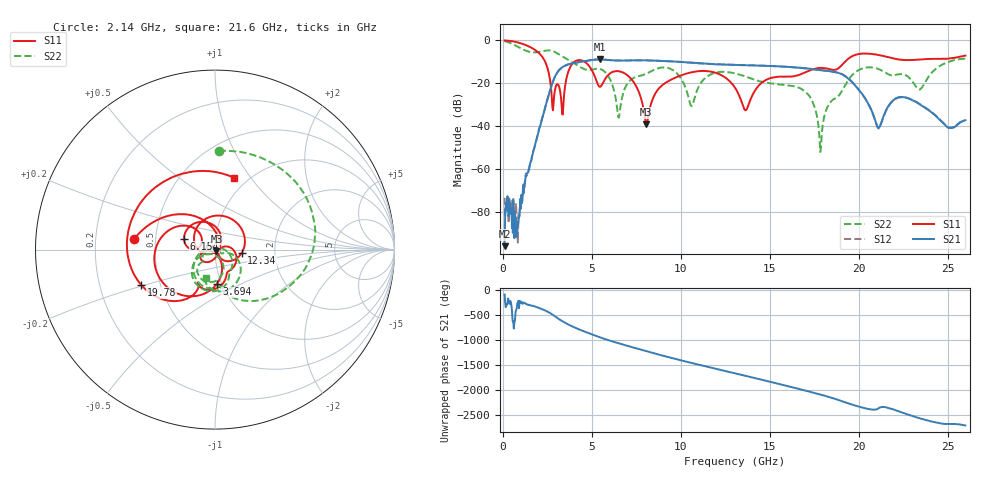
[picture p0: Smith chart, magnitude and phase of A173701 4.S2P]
!  2-Port S-parameters saved by WinCal
! VAR MeasName=S-Parameters (CALIBRATED_DATA) read from VNA (N5245A)
! VAR MeasDate=2017-6-7 10:28:41
! VAR NAME=A173701 4
! VAR FILENAME=A173701 4.S2P
! VAR DATE=2017-6-7 10:28:41
! VAR PHYS_PORTS=1,2
# Hz S DB R 50
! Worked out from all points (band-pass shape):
!   801 points, 100 MHz to 26 GHz, reference 50 ohm
!   highest |S21| = -8.86 dB at 5.442 GHz (marker M1); lowest = -96.1 dB at 100 MHz (marker M2)
!   |S21| within 3 dB of the highest: 3.481 GHz to 14.81 GHz (11.32 GHz wide, 124 % of centre)
!   lowest |S11| = -39.2 dB at 8.064 GHz (marker M3), VSWR 1.02, Z = 50.8 - j0.768 ohm
!   |S11| at or under -10 dB: 2.38 GHz to 4.019 GHz (1.639 GHz wide, 51.2 % of centre); 4.605 GHz to 19.23 GHz (14.62 GHz wide, 123 % of centre)
!   |S22| runs from -52.1 to -0.3 dB; largest |S21 - S12| = 0.0043
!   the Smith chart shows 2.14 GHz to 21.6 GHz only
!   S11 on the Smith chart (normalised r, x): 2.14 GHz: 0.38, +0.06; 3.694 GHz: 0.94, -0.38; 6.154 GHz: 0.70, +0.09; 12.34 GHz: 1.35, -0.05; 19.78 GHz: 0.39, -0.19; 21.6 GHz: 0.87, +0.83
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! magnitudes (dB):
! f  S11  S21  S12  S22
! 100 MHz  0.0  -96.1  -73.5  -0.3
! 909.4 MHz  -1.1  -82.4  -81.9  -3.2
! 2.14 GHz  -6.9  -38.6  -38.6  -5.2
! 2.82 GHz  -32.6  -19.1  -19.1  -5.0
! 3.694 GHz  -14.3  -11.1  -11.1  -9.2
! 4.438 GHz  -9.3  -9.9  -9.9  -12.8
! 5.442 GHz  -21.6  -8.9  -8.9  -13.3
! 6.154 GHz  -14.8  -9.3  -9.3  -20.7
! 6.51 GHz  -14.4  -9.4  -9.4  -36.1
! 8.064 GHz  -39.2  -9.3  -9.3  -15.5
! 8.744 GHz  -22.7  -9.5  -9.5  -13.0
! 10.62 GHz  -14.8  -10.4  -10.5  -30.6
! 12.34 GHz  -16.5  -11.2  -11.2  -14.6
! 13.05 GHz  -22.1  -11.4  -11.4  -15.4
! 13.67 GHz  -32.5  -11.5  -11.6  -16.9
! 17.39 GHz  -13.6  -13.5  -13.3  -28.3
! 17.87 GHz  -12.8  -13.9  -13.8  -50.7
! 19.78 GHz  -6.8  -20.8  -20.8  -15.0
! 21.08 GHz  -6.7  -40.7  -40.7  -13.3
! 21.6 GHz  -7.7  -31.7  -31.9  -15.5
! 21.69 GHz  -7.9  -30.4  -30.6  -15.9
! 26 GHz  -7.1  -37.3  -37.2  -8.6
